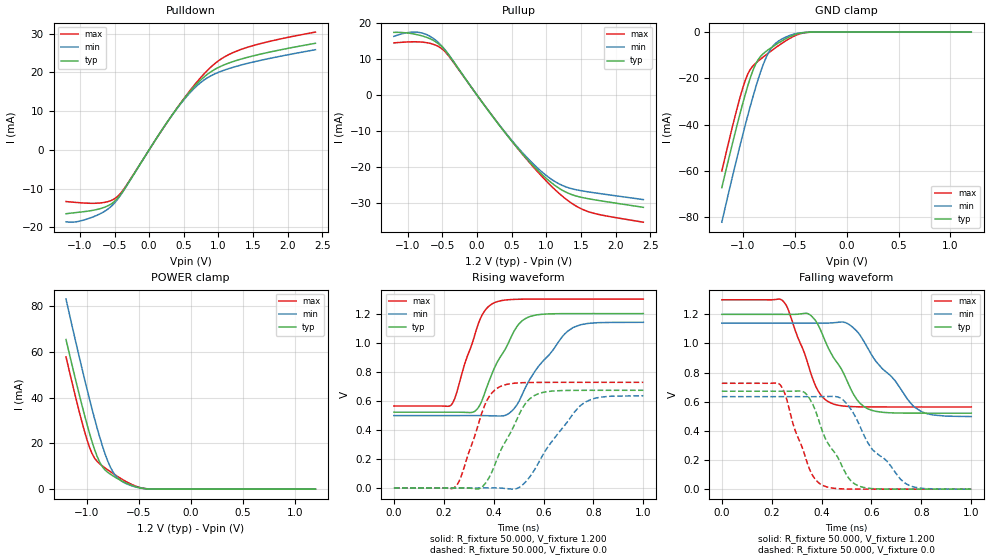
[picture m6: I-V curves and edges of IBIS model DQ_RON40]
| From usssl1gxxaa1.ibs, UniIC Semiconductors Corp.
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|   Model DQ_RON40
[Model] DQ_RON40
Model_type I/O
Vinl =  0.500V
Vinh =  0.700V
Vmeas =  0.600V
Rref =  50.000
Vref =  0.600V
C_comp   1.373pF   1.353pF   1.403pF
[Model Spec]
Vinh   0.700V   0.670V   0.750V
Vinl   0.500V   0.470V   0.550V
Vmeas   0.600V   0.570V   0.650V
Vref   0.600V   0.570V   0.650V
Rref   50.000   NA   NA
[Temperature Range]   25.000   0.125k   -40.000
[Voltage Range]   1.200V   1.140V   1.300V
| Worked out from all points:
|   slope of the pulldown table from 0 to 0.18 V, typ, clamps not added: 36 ohm
|   slope of the pullup table from 0 to 0.18 V, typ, clamps not added: 37.6 ohm
|   GND clamp passes 1 mA (typ) near -0.49 V on its own axis
|   POWER clamp passes 1 mA (typ) near -0.53 V on its own axis
|   rising waveform, R_fixture 50.000, V_fixture 1.200: 20-80 % time 112ps typ, 153ps min, 82.8ps max; typ from 0.522 V to 1.2 V
|   rising waveform, R_fixture 50.000, V_fixture 0.0: 20-80 % time 113ps typ, 153ps min, 85ps max; typ from 0 V to 0.672 V
|   falling waveform, R_fixture 50.000, V_fixture 1.200: 20-80 % time 123ps typ, 170ps min, 93ps max; typ from 1.2 V to 0.522 V
|   falling waveform, R_fixture 50.000, V_fixture 0.0: 20-80 % time 113ps typ, 158ps min, 84.3ps max; typ from 0.672 V to 0 V
[Pulldown]
|Voltage   I(typ)   I(min)   I(max)
-1.2V     -16.5mA    -18.58mA   -13.36mA
-1.015V   -16.12mA   -18.46mA   -13.64mA
-756mV    -15.42mA   -16.92mA   -13.78mA
-571mV    -14.22mA   -14.96mA   -13.24mA
-460mV    -12.61mA   -12.88mA   -12.11mA
-349mV    -9.901mA   -9.986mA   -9.712mA
354mV     9.556mA    9.483mA    9.558mA
613mV     15.55mA    15.19mA    15.84mA
798mV     18.9mA     18.1mA     19.71mA
1.02V     21.44mA    20.15mA    23.23mA
1.279V    23.17mA    21.66mA    25.61mA
2.4V      27.51mA    25.85mA    30.4mA
[Pullup]
|Voltage   I(typ)   I(min)   I(max)
-1.2V     17.52mA    16.42mA    14.6mA
-1.004V   17.34mA    17.45mA    14.85mA
-819mV    16.67mA    17.45mA    14.85mA
-634mV    15.31mA    15.87mA    14.22mA
-486mV    13.07mA    13.22mA    12.58mA
106mV     -2.836mA   -2.815mA   -2.798mA
513mV     -13.1mA    -12.88mA   -13.09mA
846mV     -20.4mA    -19.84mA   -20.77mA
1.142V    -25.44mA   -24.31mA   -26.67mA
1.364V    -27.73mA   -26.08mA   -30.15mA
1.586V    -28.82mA   -26.93mA   -32.37mA
2.4V      -31.3mA    -29.14mA   -35.44mA
[GND_clamp]
|Voltage   I(typ)   I(min)   I(max)
-1.2V     -67.26mA   -82.22mA   -60.1mA
-1.05V    -39.62mA   -53.62mA   -32.4mA
-1V       -31.05mA   -44.64mA   -24.37mA
-950mV    -23.16mA   -36.01mA   -18.1mA
-925mV    -19.62mA   -31.85mA   -16.02mA
-875mV    -13.89mA   -23.97mA   -13.48mA
-800mV    -9.288mA   -13.81mA   -10.72mA
-750mV    -7.535mA   -8.829mA   -8.993mA
-675mV    -5.274mA   -4.578mA   -6.506mA
-525mV    -1.587mA   -1.138mA   -2.208mA
-375mV    -90.13uA   -87.27uA   -132.9uA
1.2V      0A         0A         0A
[POWER_clamp]
|Voltage   I(typ)   I(min)   I(max)
-1.2V     65.51mA    83.21mA    57.91mA
-1.05V    37.38mA    53.57mA    29.99mA
-1V       28.74mA    44.18mA    21.95mA
-950mV    20.85mA    35.16mA    15.65mA
-925mV    17.34mA    30.84mA    13.56mA
-875mV    11.74mA    22.7mA     11.06mA
-800mV    7.436mA    12.47mA    8.502mA
-750mV    5.864mA    7.69mA     6.933mA
-675mV    3.901mA    3.837mA    4.735mA
-525mV    971.5uA    903.1uA    1.25mA
-400mV    85.95uA    125.9uA    91.19uA
1.2V      0A         0A         0A
[Ramp]
| variable   typ   min   max
dV/dt_r   0.403/0.113n   0.381/0.153n   0.436/85.122p
dV/dt_f   0.407/0.123n   0.385/0.170n   0.441/93.034p
R_load = 50.000
[Rising Waveform]
R_fixture= 50.000
V_fixture= 1.200
V_fixture_min= 1.140
V_fixture_max= 1.300
|time   V(typ)   V(min)   V(max)
0s        521.6mV    498.1mV    564.2mV
229ps     521.7mV    498.1mV    570.4mV
331ps     537.9mV    498.2mV    1.093V
363ps     648.1mV    497.8mV    1.217V
404ps     830mV      496mV      1.276V
467ps     1.028V     520.8mV    1.296V
520ps     1.158V     665mV      1.299V
578ps     1.192V     834mV      1.3V
718ps     1.2V       1.104V     1.3V
1ns       1.2V       1.14V      1.3V
[Rising Waveform]
R_fixture= 50.000
V_fixture= 0.0
V_fixture_min= 0.0
V_fixture_max= 0.0
|time   V(typ)   V(min)   V(max)
0s        38.4nV     662.6nV    22.61nV
243ps     103.7uV    -5.875uV   3.668mV
268ps     364.3uV    -18.19uV   72.4mV
350ps     2.457mV    170.5uV    503.2mV
383ps     75.89mV    422.5uV    631.9mV
430ps     265.3mV    -968.6uV   700.7mV
503ps     509.9mV    4.462mV    723.6mV
577ps     647.2mV    165mV      726.5mV
764ps     672.1mV    588.5mV    726.9mV
1ns       672.2mV    634.8mV    726.9mV
[Falling Waveform]
R_fixture= 50.000
V_fixture= 1.200
V_fixture_min= 1.140
V_fixture_max= 1.300
|time   V(typ)   V(min)   V(max)
0s        1.2V       1.14V      1.3V
243ps     1.2V       1.14V      1.295V
269ps     1.2V       1.14V      1.219V
359ps     1.189V     1.14V      784.1mV
394ps     1.1V       1.14V      653mV
446ps     907.8mV    1.142V     585.2mV
508ps     720.5mV    1.133V     567.8mV
584ps     552.6mV    970.9mV    564.6mV
774ps     521.8mV    561.1mV    564.2mV
1ns       521.6mV    498.3mV    564.2mV
[Falling Waveform]
R_fixture= 50.000
V_fixture= 0.0
V_fixture_min= 0.0
V_fixture_max= 0.0
|time   V(typ)   V(min)   V(max)
0s        672.2mV    635mV      726.9mV
233ps     672.1mV    635mV      718.1mV
334ps     659.9mV    634.8mV    225.1mV
364ps     583.9mV    634.8mV    93.81mV
403ps     398.3mV    635.3mV    27.25mV
485ps     146.7mV    614.3mV    1.927mV
552ps     19.66mV    438.3mV    218.4uV
598ps     4.574mV    284.1mV    48.34uV
736ps     56.59uV    39.44mV    548.9nV
1ns       48.27nV    18.32uV    18.02nV
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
